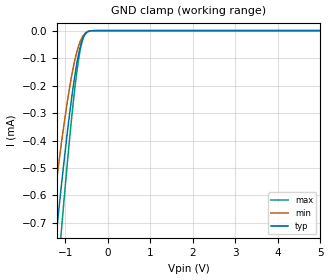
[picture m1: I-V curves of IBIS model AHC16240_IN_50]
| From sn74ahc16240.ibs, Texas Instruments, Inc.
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[Model]   AHC16240_IN_50
Model_type  Input
Vinl = 1.575
Vinh = 3.85
| variable   typ   min   max
C_comp   0.83pF   0.75pF   0.92pF
[Temperature Range]   40   100   -40
| Ambient temperature   25   85   -40
[Voltage range]   5   4.5   5.5
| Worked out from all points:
|   GND clamp passes 1 mA (typ) near -1.38 V on its own axis
[GND Clamp]
| AHC16240_IN_50
|   Voltage   I(typ)   I(min)   I(max)
-5.5V     -8.851mA   -7.354mA   -10.02mA
-1.37V    -983.1uA   -749.2uA   -1.247mA
-1.315V   -896.4uA   -678.6uA   -1.141mA
-1.21V    -734.8uA   -547.4uA   -941.1uA
-1.11V    -586.6uA   -428.2uA   -755.8uA
-1.085V   -550.6uA   -399.5uA   -710.3uA
-905mV    -308.2uA   -210.9uA   -399.5uA
-810mV    -197.4uA   -130.2uA   -253.9uA
-730mV    -118.5uA   -76.84uA   -149uA
-610mV    -36.66uA   -25.92uA   -41.55uA
-480mV    -4.927uA   -3.935uA   -4.07uA
5V        7.166nA    474.1pA    66.12nA
